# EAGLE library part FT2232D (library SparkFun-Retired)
USB to USART/FIFO/JTAG/SPI/I2C
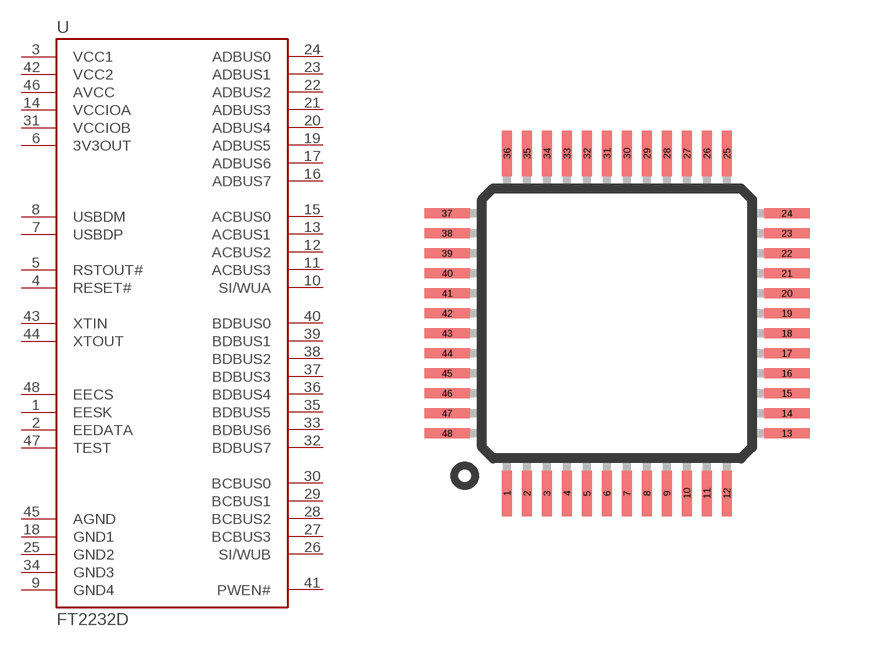
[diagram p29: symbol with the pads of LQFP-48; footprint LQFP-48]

Designator prefix -

## FT2232D  [LQFP-48]
1  EESK
2  EEDATA
3  VCC1  pwr
4  RESET#
5  RSTOUT#
6  3V3OUT  out
7  USBDP
8  USBDM
9  GND4
10  SI/WUA
11  ACBUS3
12  ACBUS2
13  ACBUS1
14  VCCIOA  pwr
15  ACBUS0
16  ADBUS7
17  ADBUS6
18  GND1  pwr
19  ADBUS5
20  ADBUS4
21  ADBUS3
22  ADBUS2
23  ADBUS1
24  ADBUS0
25  GND2  pwr
26  SI/WUB
27  BCBUS3
28  BCBUS2
29  BCBUS1
30  BCBUS0
31  VCCIOB
32  BDBUS7  in
33  BDBUS6  in
34  GND3  pwr
35  BDBUS5  in
36  BDBUS4  out
37  BDBUS3  in
38  BDBUS2  out
39  BDBUS1  in
40  BDBUS0  out
41  PWEN#
42  VCC2  pwr
43  XTIN
44  XTOUT
45  AGND  pwr
46  AVCC
47  TEST  in
48  EECS

## Footprint LQFP-48 (pad centres in mm)
smd 0.254 x 1.143: 1 -2.75,-4.25; 2 -2.25,-4.25; 3 -1.75,-4.25; 4 -1.25,-4.25; 5 -0.75,-4.25; 6 -0.25,-4.25; 7 0.25,-4.25; 8 0.75,-4.25; 9 1.25,-4.25; 10 1.75,-4.25; 11 2.25,-4.25; 12 2.75,-4.25; 25 2.75,4.25; 26 2.25,4.25; 27 1.75,4.25; 28 1.25,4.25; 29 0.75,4.25; 30 0.25,4.25; 31 -0.25,4.25; 32 -0.75,4.25; 33 -1.25,4.25; 34 -1.75,4.25; 35 -2.25,4.25; 36 -2.75,4.25
smd 1.143 x 0.254: 13 4.25,-2.75; 14 4.25,-2.25; 15 4.25,-1.75; 16 4.25,-1.25; 17 4.25,-0.75; 18 4.25,-0.25; 19 4.25,0.25; 20 4.25,0.75; 21 4.25,1.25; 22 4.25,1.75; 23 4.25,2.25; 24 4.25,2.75; 37 -4.25,2.75; 38 -4.25,2.25; 39 -4.25,1.75; 40 -4.25,1.25; 41 -4.25,0.75; 42 -4.25,0.25; 43 -4.25,-0.25; 44 -4.25,-0.75; 45 -4.25,-1.25; 46 -4.25,-1.75; 47 -4.25,-2.25; 48 -4.25,-2.75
